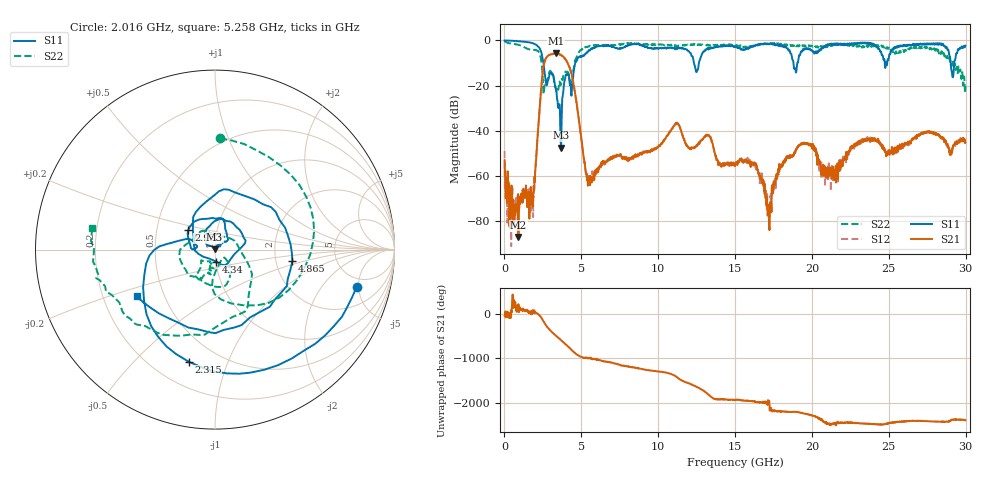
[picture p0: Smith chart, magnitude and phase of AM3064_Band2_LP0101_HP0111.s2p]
# Hz S DB R 50.0
!freq dBS11 angS11 dBS21 angS21 dBS12 angS12 dBS22 angS22
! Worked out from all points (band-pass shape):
!   1600 points, 10 MHz to 29.98 GHz, reference 50 ohm
!   highest |S21| = -5.72 dB at 3.346 GHz (marker M1); lowest = -87.1 dB at 909.7 MHz (marker M2)
!   |S21| within 3 dB of the highest: 2.647 GHz to 4.005 GHz (1.358 GHz wide, 40.8 % of centre)
!   lowest |S11| = -47.5 dB at 3.684 GHz (marker M3), VSWR 1.01, Z = 49.7 + j0.336 ohm
!   |S11| at or under -10 dB: 2.536 GHz to 4.595 GHz (2.059 GHz wide, 57.7 % of centre); 12.32 GHz to 12.65 GHz (326.2 MHz wide, 2.61 % of centre); 18.8 GHz to 19.05 GHz (250 MHz wide, 1.32 % of centre)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
!   |S22| runs from -23.8 to -0.2 dB; largest |S21 - S12| = 0.018
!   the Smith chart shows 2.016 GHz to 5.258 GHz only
!   S11 on the Smith chart (normalised r, x): 2.016 GHz: 3.85, -4.76; 2.315 GHz: 0.35, -0.73; 2.953 GHz: 0.73, +0.17; 4.34 GHz: 1.00, -0.13; 4.865 GHz: 2.47, -0.39; 5.258 GHz: 0.35, -0.24
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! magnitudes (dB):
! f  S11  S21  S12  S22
! 10 MHz  0.0  -53.1  -48.9  -0.2
! 909.7 MHz  -0.4  -87.1  -71.4  -2.0
! 1.753 GHz  -1.1  -69.4  -68.5  -4.2
! 2.016 GHz  -1.8  -56.9  -57.9  -4.1
! 2.315 GHz  -3.9  -27.7  -27.6  -6.6
! 2.953 GHz  -14.7  -6.4  -6.3  -13.5
! 3.346 GHz  -21.9  -5.7  -5.9  -21.8
! 3.684 GHz  -47.5  -6.6  -6.4  -18.3
! 4.34 GHz  -23.5  -14.4  -14.1  -22.0
! 4.865 GHz  -7.2  -36.5  -36.4  -5.0
! 5.015 GHz  -7.4  -44.5  -44.1  -4.3
! 5.258 GHz  -5.9  -56.6  -57.5  -3.2
! 10 GHz  -3.5  -46.9  -47.1  -1.8
! 11.24 GHz  -3.6  -36.7  -36.6  -2.6
! 15 GHz  -2.6  -54.7  -54.7  -2.0
! 16.3 GHz  -2.1  -55.0  -55.1  -2.2
! 17.22 GHz  -1.4  -81.0  -76.7  -1.5
! 18.02 GHz  -2.5  -56.2  -56.0  -1.9
! 19.99 GHz  -4.3  -47.0  -46.9  -2.3
! 21.38 GHz  -1.4  -57.0  -57.0  -2.2
! 25 GHz  -7.9  -49.3  -49.1  -3.2
! 29.98 GHz  -2.3  -45.2  -45.3  -20.2
